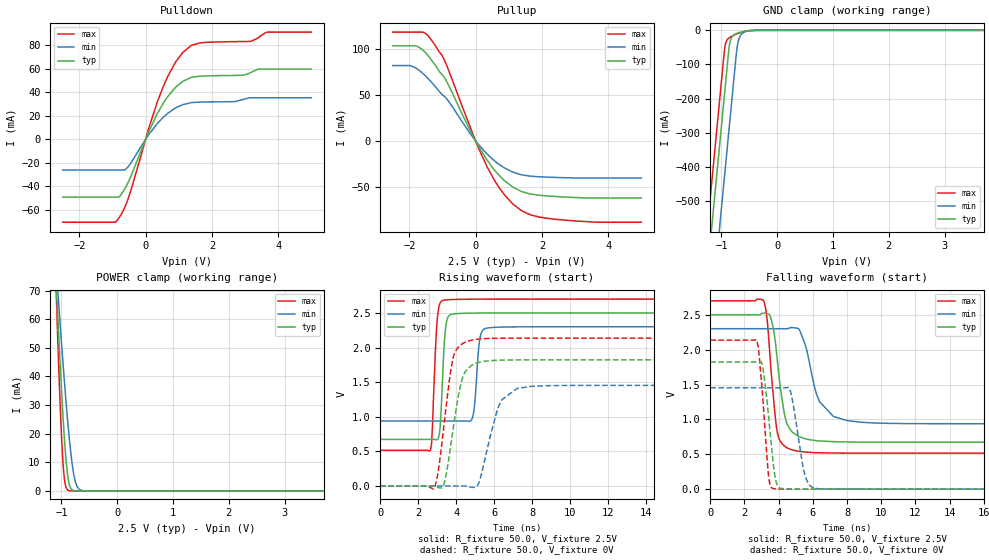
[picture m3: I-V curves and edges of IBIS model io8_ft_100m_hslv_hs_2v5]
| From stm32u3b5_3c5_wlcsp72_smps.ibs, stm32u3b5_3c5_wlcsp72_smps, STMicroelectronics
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[Model]   io8_ft_100m_hslv_hs_2v5
Model_type I/O
Polarity   Non-Inverting
Enable   Active-Low
| CAP_THRESHOLD on pad IOFT is "UDTCAPC" :
| Rising=30.0% of vddiom   Falling=70.0% of vddiom
| C_comp min and max val. don't necessarily correlate with the min and max pvt
| but are the smallest and greatest pad capacitance found.
| var   typ   min   max
C_comp   3.68195pF  3.67098pF  3.72549pF
|C_comp_pullup   2.08738pF  2.19381pF  2.32565pF
|C_comp_pulldown   1.59457pF  1.47718pF  1.39984pF
Vinl = 1.15V
Vinh = 1.35V
Vmeas = 1.25V   | Reference voltage for timing measurements
Cref  = 50.0pF   | Timing specification test load capacitance value
Rref  = 1.0MOhm   | Timing specification test load resistance value
Vref  = 1.375V   | Timing specification test load voltage
[Model Spec]
| TIME_THRESHOLD on pin ZIV11 is "CMOS" :
| Rising=50.0% of vdd   Falling=50.0% of vdd
Vinl 981.50000mV 911.50000mV 1.04650V
Vinh 1.42350V 1.31650V 1.50350V
| variable   typ   min   max
[Temperature Range] 25.0 130.0 -40.0
| variable   typ   min   max
[Voltage Range] 2.5V 2.3V 2.7V
| variable   typ   min   max
[POWER Clamp Reference] 2.5V 2.3V 2.7V
| variable   typ   min   max
[GND Clamp Reference] 0V 0V 0V
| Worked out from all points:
|   slope of the pulldown table from 0 to 0.375 V, typ, clamps not added: 16.4 ohm
|   slope of the pullup table from 0 to 0.375 V, typ, clamps not added: 16.7 ohm
|   GND clamp passes 1 mA (typ) near -0.50 V on its own axis
|   POWER clamp passes 1 mA (typ) near -0.83 V on its own axis
|   rising waveform, R_fixture 50.0, V_fixture 2.5V: 20-80 % time 197ps typ, 217ps min, 201ps max; typ from 0.673 V to 2.5 V
|   falling waveform, R_fixture 50.0, V_fixture 2.5V: 20-80 % time 580ps typ, 954ps min, 454ps max; typ from 2.5 V to 0.673 V
|   rising waveform, R_fixture 50.0, V_fixture 0V: 20-80 % time 637ps typ, 827ps min, 576ps max; typ from 0 V to 1.82 V
|   falling waveform, R_fixture 50.0, V_fixture 0V: 20-80 % time 461ps typ, 565ps min, 392ps max; typ from 1.82 V to 0 V
[POWER Clamp]
-2.5V     736.6mA    513.9mA    1.064A
-1.1V     75.38mA    79.63mA    73.18mA
-1.09V    71.2mA     76.8mA     67.14mA
-1.08V    67.05mA    73.98mA    61.2mA
-1.06V    58.89mA    68.38mA    49.67mA
-1.02V    43.22mA    57.4mA     28.67mA
-980mV    28.81mA    46.77mA    12.28mA
-940mV    16.45mA    36.61mA    3.257mA
-880mV    4.35mA     22.67mA    225.4uA
-770mV    97.5uA     4.87mA     1.193uA
-630mV    518.5nA    149.1uA    1.636nA
5V        0A         0A         0A
[GND Clamp]
-2.5V     -2.831A    -3.071A    -2.699A
-1.46V    -1.063A    -1.303A    -931.1mA
-1.21V    -637.8mA   -878.3mA   -506.1mA
-950mV    -195.8mA   -436.3mA   -64.07mA
-940mV    -178.8mA   -419.3mA   -50.67mA
-910mV    -127.8mA   -368.3mA   -31.36mA
-850mV    -37.25mA   -266.3mA   -20.72mA
-750mV    -10.68mA   -96.33mA   -12.3mA
-710mV    -8.126mA   -41.01mA   -9.515mA
-670mV    -6.142mA   -18.5mA    -7.051mA
-470mV    -612.4uA   -1.154mA   -431uA
5V        1.687nA    211.8nA    737.8pA
| variable   typ   min   max
[Pullup Reference] 2.5V 2.3V 2.7V
| variable   typ   min   max
[Pulldown Reference] 0V 0V 0V
[Pullup]
-2.5V     103.9mA    82.33mA    118.9mA
-1.98V    103.9mA    82.23mA    118.9mA
-1.74V    103mA      78.1mA     118.9mA
-1.5V     95.96mA    70.63mA    117.1mA
-1.21V    82.39mA    59.12mA    104mA
-890mV    66.01mA    46.86mA    84.06mA
-170mV    11.87mA    8.299mA    15.68mA
350mV     -21.19mA   -14.53mA   -28.53mA
850mV     -42.77mA   -29.12mA   -58.03mA
1.38V     -55.27mA   -37.08mA   -76.15mA
2.5V      -60.98mA   -40.04mA   -86.01mA
5V        -62.43mA   -40.58mA   -88.86mA
[Pulldown]
-2.5V     -49.09mA   -26.02mA   -70.37mA
-920mV    -49.09mA   -26.02mA   -70.37mA
-830mV    -49.09mA   -26.02mA   -67.8mA
-510mV    -35.57mA   -22.69mA   -49.05mA
90mV      6.138mA    3.798mA    8.848mA
520mV     30.1mA     18.41mA    43.96mA
940mV     45.18mA    27.25mA    67.1mA
1.38V     52.7mA     31.24mA    79.88mA
2.68V     54.32mA    32.09mA    83.06mA
3.2V      57.2mA     35.33mA    83.52mA
3.67V     59.71mA    35.33mA    91.16mA
5V        59.71mA    35.33mA    91.17mA
[Ramp]
dV/dt_r 1.09344V/636.18338ps 871.7827mV/823.14411ps 1.28161V/575.20294ps
dV/dt_f 1.09609V/578.46842ps 816.98961mV/880.21492ps 1.31053V/452.05822ps
R_load = 50.0
| Removed startup time: 0s 0s 0s  .
| Removed end time: 19.25ns.
[Rising Waveform]
R_fixture   = 50.0
V_fixture   = 2.5V
V_fixture_min = 2.3V
V_fixture_max = 2.7V
0s        673.2mV    938.3mV    515.8mV
2.65ns    673.2mV    938.3mV    527mV
3ns       668.4mV    938.4mV    2.406V
3.25ns    1.368V     938.3mV    2.676V
3.4ns     2.175V     938.4mV    2.686V
3.55ns    2.43V      938.4mV    2.69V
4.85ns    2.497V     981.6mV    2.698V
5.25ns    2.498V     2.139V     2.699V
5.55ns    2.499V     2.277V     2.699V
19.25ns   2.5V       2.3V       2.7V
| Removed startup time: 0s 0s 0s  .
| Removed end time: 39.25ns.
[Falling Waveform]
R_fixture   = 50.0
V_fixture   = 2.5V
V_fixture_min = 2.3V
V_fixture_max = 2.7V
0s        2.5V       2.3V       2.7V
3.1ns     2.522V     2.3V       2.71V
3.55ns    2.445V     2.3V       1.715V
3.9ns     1.902V     2.3V       845.9mV
4.35ns    1.064V     2.3V       615.9mV
4.8ns     818.3mV    2.317V     562.2mV
5.55ns    722.6mV    2.075V     532mV
6.4ns     691.3mV    1.253V     521.6mV
8ns       676.5mV    983.5mV    516.8mV
39.25ns   673.2mV    938.4mV    515.8mV
| Removed startup time: 0s 0s 0s  .
| Removed end time: 39.2ns.
[Rising Waveform]
R_fixture   = 50.0
V_fixture   = 0V
V_fixture_min = 0V
V_fixture_max = 0V
0s        5.238nV    85.5nV     4.322nV
2.85ns    -168.3uV   -218.7nV   -26.27mV
3.35ns    23.57mV    -4.579uV   867mV
3.85ns    849.1mV    -15.72uV   1.865V
4.3ns     1.533V     -142.6uV   2.051V
4.9ns     1.756V     -21.01mV   2.112V
5.25ns    1.79V      93.78mV    2.124V
6.3ns     1.817V     1.191V     2.134V
7.2ns     1.821V     1.409V     2.135V
39.2ns    1.822V     1.453V     2.136V
| Removed startup time: 0s 0s 0s  .
| Removed end time: 19.25ns.
[Falling Waveform]
R_fixture   = 50.0
V_fixture   = 0V
V_fixture_min = 0V
V_fixture_max = 0V
0s        1.822V     1.453V     2.136V
2.7ns     1.823V     1.453V     2.142V
3.1ns     1.702V     1.453V     1.212V
3.4ns     1.071V     1.453V     212.2mV
3.65ns    448mV      1.453V     11.4mV
3.95ns    44.67mV    1.453V     3.984mV
4.65ns    3.322mV    1.432V     1.93mV
5.5ns     1.451mV    239.1mV    897.3uV
5.95ns    974.2uV    28.87mV    605.6uV
19.25ns   5.191uV    19.17uV    1.586uV
